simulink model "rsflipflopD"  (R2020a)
settings: Solver=ode45  StartTime=0.0  StopTime=Inf  FixedStep=1  RelTol=1e-3  EnableMultiTasking=on

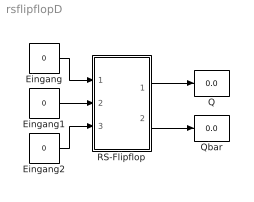
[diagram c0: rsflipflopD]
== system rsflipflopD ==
  note: .
  Eingang : Constant  Value=0  OutDataTypeStr=double
  Eingang1 : Constant  Value=0  OutDataTypeStr=double
  Eingang2 : Constant  Value=0  OutDataTypeStr=double
  Q : Display
  Qbar : Display
  RS-Flipflop : Subsystem  mask(RSFlipFlop){initial_condition=0}
      mask prompts: initial_condition "Initial condition"
      mask help: getriggertes R-S-Flip-Flop
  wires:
  RS-Flipflop/1(Q) -> Q/1
  RS-Flipflop/2(!Q) -> Qbar/1
  Eingang/1 -> RS-Flipflop/1(S)
  Eingang1/1 -> RS-Flipflop/2(CLK)
  Eingang2/1 -> RS-Flipflop/3(R)

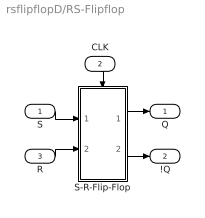
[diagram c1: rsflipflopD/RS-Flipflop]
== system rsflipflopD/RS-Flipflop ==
  S : Inport
  CLK : Inport  Port=2
  R : Inport  Port=3
  S-R-Flip-Flop : Subsystem
  Q : Outport
  !Q : Outport  Port=2
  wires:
  CLK/1 -> S-R-Flip-Flop/Trigger
  S/1 -> S-R-Flip-Flop/1(S)
  S-R-Flip-Flop/1(Q) -> Q/1
  R/1 -> S-R-Flip-Flop/2(R)
  S-R-Flip-Flop/2(!Q) -> !Q/1

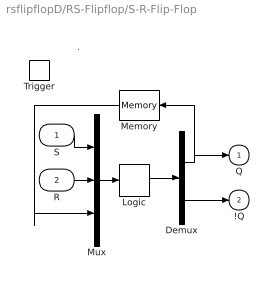
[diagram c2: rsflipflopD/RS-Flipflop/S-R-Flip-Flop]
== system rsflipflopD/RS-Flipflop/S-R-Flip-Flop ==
  note: .
  S : Inport
  R : Inport  Port=2
  Trigger : TriggerPort  TriggerType=falling  VariantControl=Variant  StatesWhenEnabling=reset
  Demux : Demux  Outputs=2
  Logic : CombinatorialLogic  TruthTable=[0 1; 1 0; 0 1; 0 1; 1 0; 1 0; 0 0; 0 0]
  Memory : Memory  InitialCondition=initial_condition  InheritSampleTime=on
  Mux : Mux  Inputs=3
  Q : Outport  InitialOutput=0
  !Q : Outport  Port=2  InitialOutput=1
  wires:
  Memory/1 -> Mux/3
  Mux/1 -> Logic/1
  Logic/1 -> Demux/1
  Demux/2 -> !Q/1
  Demux/1 -> Q/1, Memory/1
  S/1 -> Mux/1
  R/1 -> Mux/2
